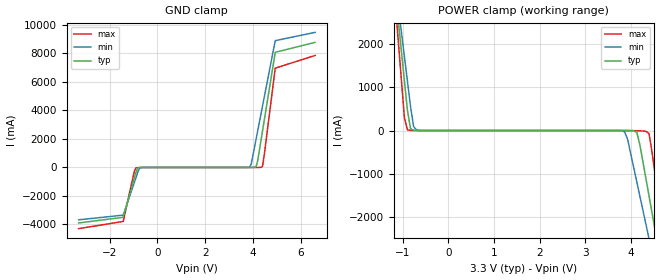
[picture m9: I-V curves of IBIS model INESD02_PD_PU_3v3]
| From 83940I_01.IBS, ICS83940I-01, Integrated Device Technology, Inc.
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[Model] INESD02_PD_PU_3v3
Model_type  Input
Polarity   Non-Inverting
Vinl = 0.8V
Vinh = 2.0V
|   typ   min   max
C_comp   2pF   1.5pF   2.5pF
|   typ   min   max
[Voltage range]   3.3V   3.15V   3.45V
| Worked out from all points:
|   GND clamp passes 1 mA (typ) near -0.59 V on its own axis
|   POWER clamp passes 1 mA (typ) near -0.70 V on its own axis
[GND_clamp]
-3.3V     -3.894A    -3.674A    -4.294A
-1.433V   -3.498A    -3.345A    -3.788A
-963.9mV  -730.3mA   -1.043A    -250mA
-896.9mV  -335.4mA   -714.8mA   -27.09mA
-695.9mV  -3.422mA   -10.72mA   -6.487mA
3.861V    132.6uA    27.79mA    76.29uA
3.928V    264.4uA    239.1mA    80.1uA
4.129V    40.53mA    1.967A     342uA
4.196V    445.9mA    2.544A     962.5uA
4.397V    2.525A     4.275A     64.09mA
4.933V    8.079A     8.897A     6.966A
6.6V      8.773A     9.475A     7.854A
[POWER_clamp]
-3.3V     6.7A       6.327A     7.39A
-1.165V   3.23A      3.44A      2.951A
-1.031V   1.843A     2.286A     1.176A
-963.9mV  1.149A     1.709A     289.6mA
-896.9mV  456.5mA    1.133A     15.41mA
-695.9mV  812.8uA    10.76mA    565.7uA
3.861V    -638.5uA   -26.24mA   -108.3uA
4.129V    -41.93mA   -1.19A     -4.977mA
4.33V     -1.119A    -2.176A    -17.94mA
4.531V    -2.305A    -3.163A    -1.019A
4.732V    -3.492A    -4.151A    -2.536A
6.6V      -5.075A    -5.469A    -4.558A
